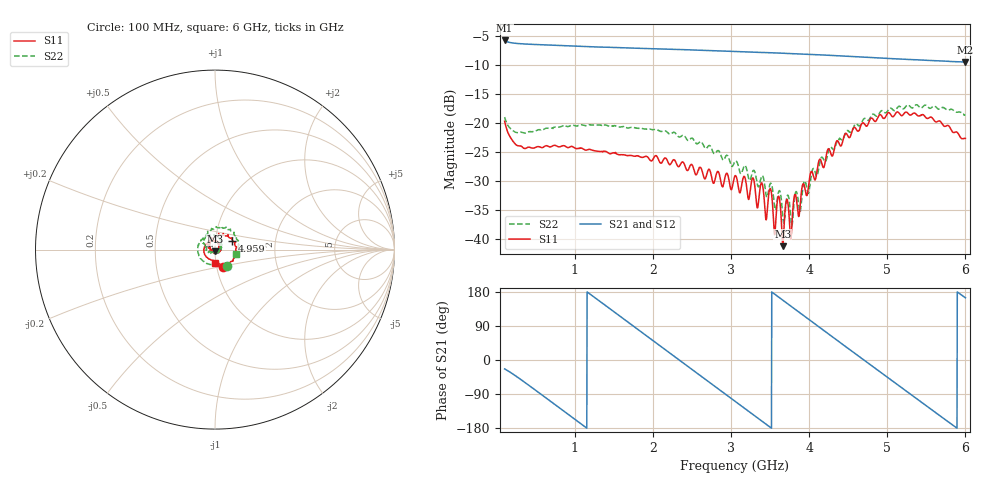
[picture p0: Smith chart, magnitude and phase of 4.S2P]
!Agilent Technologies,E5071C,MY46316741,A.11.02
!Date: Thu Dec 16 09:42:44 2021
!Data & Calibration Information:
!Freq	S11:SOLT4(ON)	S21:SOLT4(ON)	S12:SOLT4(ON)	S22:SOLT4(ON)
!PortZ  Port1:50+j0  Port2:50+j0
!Above PortZ is port z conversion or system Z0 setting when saving the data.
!When reading, reference impedance value at option line is always used.
# Hz S dB R 50
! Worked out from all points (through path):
!   1593 points, 100 MHz to 6 GHz, reference 50 ohm
!   highest |S21| = -5.77 dB at 100 MHz (marker M1); lowest = -9.5 dB at 6 GHz (marker M2)
!   group delay of S21, straight-line fit = 422 ps
!   lowest |S11| = -41.2 dB at 3.661 GHz (marker M3), VSWR 1.02, Z = 50.1 - j0.861 ohm
!   |S11| at or under -10 dB: start of sweep to end of sweep
!   |S22| runs from -37.7 to -16.8 dB; largest |S21 - S12| = 0.0027
!   S11 on the Smith chart (normalised r, x): 100 MHz: 1.07, -0.20; 4.959 GHz: 1.21, +0.12; 6 GHz: 0.99, -0.15
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1e8  -19.68 -65.6  -5.77 -23.5  -5.77 -23.5  -18.96 -53.7
5.92902e8  -24.18 -134.6  -6.53 -94.5  -6.53 -94.4  -21.13 -116.5
1.085804e9  -24.30 167.5  -6.78 -169.6  -6.79 -169.6  -20.29 -171.8
1.619472e9  -25.45 124.1  -7.03 109.1  -7.03 109.2  -20.58 144.3
2.067902e9  -26.16 97.4  -7.22 40.9  -7.22 41.0  -21.21 110.6
2.486683e9  -27.12 60.5  -7.40 -23.0  -7.41 -23.0  -22.62 75.0
3.05e9  -29.07 21.0  -7.67 -108.9  -7.68 -108.7  -26.61 33.7
3.390955e9  -30.28 -14.6  -7.84 -160.7  -7.84 -160.5  -29.14 1.5
3.450251e9  -36.65 -28.6  -7.86 -169.8  -7.87 -169.6  -32.52 0.4
3.502136e9  -31.26 -34.4  -7.89 -177.7  -7.90 -177.5  -30.39 -17.7
3.557726e9  -39.22 -49.3  -7.91 173.8  -7.92 174.0  -34.46 -16.5
3.609611e9  -32.59 -63.4  -7.95 165.9  -7.95 166.1  -31.77 -42.4
3.661495e9  -41.19 -80.0  -7.97 158.0  -7.98 158.1  -36.14 -36.5
3.709673e9  -33.22 -104.7  -8.00 150.6  -8.01 150.8  -33.09 -76.1
3.765264e9  -39.98 -123.6  -8.03 142.2  -8.04 142.3  -36.52 -68.1
3.813442e9  -32.33 -143.3  -8.06 134.8  -8.07 135.0  -32.83 -111.8
4.035804e9  -28.38 166.2  -8.19 101.0  -8.19 101.2  -28.34 -160.7
4.539824e9  -21.81 77.7  -8.52 24.2  -8.52 24.4  -21.51 131.0
4.958606e9  -19.20 27.4  -8.83 -39.1  -8.83 -38.9  -18.10 85.5
5.017902e9  -18.19 20.3  -8.87 -48.1  -8.87 -47.9  -17.65 75.5
5.436683e9  -18.57 -31.9  -9.14 -111.3  -9.13 -111.0  -17.38 35.6
6e9  -22.64 -91.2  -9.48 164.1  -9.47 164.4  -18.55 -11.8
